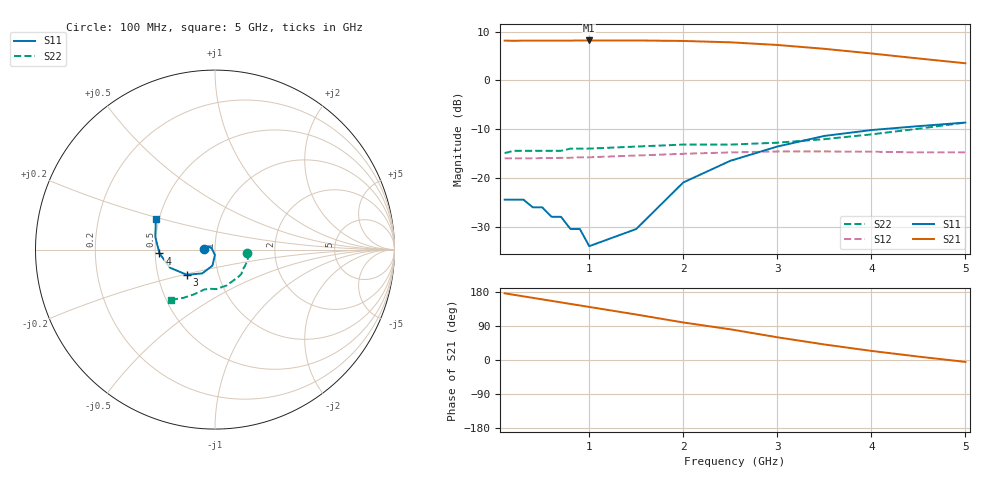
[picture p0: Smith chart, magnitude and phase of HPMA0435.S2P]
! HPMA-0435
! Typical S-Parameters, Z  = 50 , T  = 25 C, I  = 25mA
# ghz s ma r 50
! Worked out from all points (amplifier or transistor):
!   18 points, 100 MHz to 5 GHz, reference 50 ohm
!   highest |S21| = 8.2 dB at 1 GHz (marker M1)
!   |S21| within 3 dB of that: start of sweep to 4.162 GHz
!   unconditionally stable (mu >= 1): start of sweep to end of sweep
!   at 400 MHz: K = 1.38, MAG = 8.4 dB, |S12| = -16.0 dB
!   at 1 GHz: K = 1.35, MAG = 8.4 dB, |S12| = -15.8 dB
!   at 5 GHz: K = 1.38, MAG = 5.4 dB, |S12| = -14.8 dB
!   S11 on the Smith chart (normalised r, x): 100 MHz: 0.89, +0.01; 3 GHz: 0.70, -0.21; 4 GHz: 0.53, -0.03; 5 GHz: 0.48, +0.19
0.1  0.06 177.0  2.56 176.0  0.159 0.0  0.18 -6.0
0.2  0.06 173.0  2.55 172.0  0.159 0.0  0.19 -11.0
0.3  0.06 170.0  2.56 168.0  0.159 1.0  0.19 -17.0
0.4  0.05 166.0  2.56 164.0  0.159 1.0  0.19 -22.0
0.5  0.05 162.0  2.56 160.0  0.16 1.0  0.19 -28.0
0.6  0.04 160.0  2.56 156.0  0.16 1.0  0.19 -33.0
0.7  0.04 157.0  2.56 152.0  0.161 2.0  0.19 -38.0
0.8  0.03 155.0  2.56 148.0  0.161 2.0  0.2 -42.0
0.9  0.03 154.0  2.57 144.0  0.163 2.0  0.2 -48.0
1  0.02 157.0  2.57 140.0  0.163 2.0  0.2 -52.0
1.5  0.03 -91.0  2.57 120.0  0.17 2.0  0.21 -72.0
2  0.09 -99.0  2.54 99.0  0.177 1.0  0.22 -88.0
2.5  0.15 -118.0  2.46 81.0  0.183 1.0  0.22 -97.0
3  0.21 -138.0  2.31 60.0  0.187 -2.0  0.23 -105.0
3.5  0.27 -158.0  2.11 41.0  0.187 -5.0  0.25 -110.0
4  0.31 -176.0  1.89 24.0  0.186 -7.0  0.28 -116.0
4.5  0.34 168.0  1.68 9.0  0.183 -8.0  0.32 -123.0
5  0.37 153.0  1.5 -5.0  0.183 -9.0  0.37 -131.0
